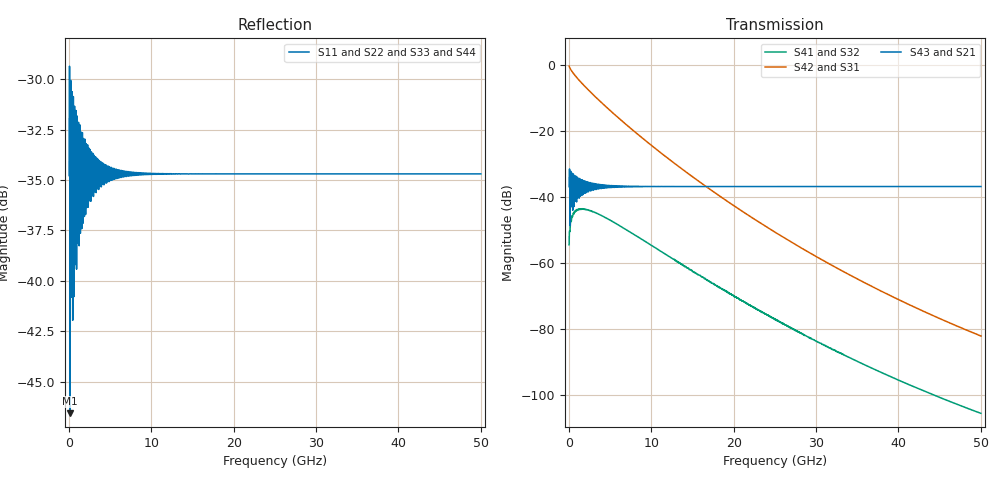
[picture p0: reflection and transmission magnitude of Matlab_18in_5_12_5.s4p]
! Generated by program util_convert_matmxmd4pspars_to_s4psended on 02-09-2011 12:57:13
!  1 ----xxxxxxxxxxxxxxxxxx---- 3
!  xxxxxxxxxxxxxxxxxx
!  (Input) xxxxxxxxxxxxxxxxxx  (Output)
!  xxxxxxxxxxxxxxxxxx
!  2 ----xxxxxxxxxxxxxxxxxx---- 4
# MHZ S DB R 50.00
! FREQ  S11  S12  S13  S14
!  S21  S22  S23  S24
!  S31  S32  S33  S34
!  S41  S42  S43  S44
!  DB  ANG  DB  ANG  DB  ANG  DB  ANG
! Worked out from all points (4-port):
!   2048 points, 24.41 MHz to 50 GHz, reference 50 ohm
!   strongest paths, dB at 24.41 MHz, 12.52 GHz, 25.02 GHz, 37.52 GHz, 50 GHz:
!     S43: -36.9, -36.8, -36.8, -36.8, -36.8
!     S21: -36.9, -36.8, -36.8, -36.8, -36.8
!     S42: -0.4, -29.3, -50.7, -68.0, -82.1
!     S31: -0.4, -29.3, -50.7, -68.0, -82.1
!     S41: -54.5, -58.6, -77.2, -92.7, -105.5
!     S32: -54.5, -58.6, -77.2, -92.7, -105.5
!   lowest |S11| = -46.6 dB at 146.5 MHz (marker M1), VSWR 1.01, Z = 49.6 + j0.208 ohm
!   |S11| at or under -10 dB: start of sweep to end of sweep
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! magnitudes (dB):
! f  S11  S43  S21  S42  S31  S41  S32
! 24.41 MHz  -34.8  -36.9  -36.9  -0.4  -0.4  -54.5  -54.5
! 146.5 MHz  -46.6  -48.7  -48.7  -1.1  -1.1  -49.7  -49.7
! 903.3 MHz  -36.1  -38.3  -38.3  -3.7  -3.7  -44.3  -44.3
! 3.271 GHz  -35.2  -37.3  -37.3  -9.8  -9.8  -44.8  -44.8
! 27.29 GHz  -34.7  -36.8  -36.8  -54.1  -54.1  -80.1  -80.1
! 42.97 GHz  -34.7  -36.8  -36.8  -74.5  -74.5  -98.6  -98.6
! 50 GHz  -34.7  -36.8  -36.8  -82.1  -82.1  -105.5  -105.5
